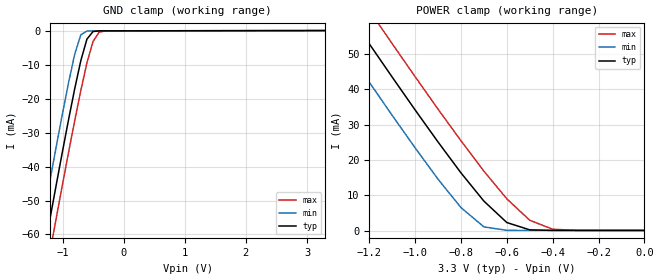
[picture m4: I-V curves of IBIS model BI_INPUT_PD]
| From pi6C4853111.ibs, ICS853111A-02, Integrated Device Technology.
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[Model]   BI_INPUT_PD
Model_type   Input
Polarity   Non-Inverting
Vinl = 1.4V
Vinh = 1.85V
|   typ   min   max
C_comp   2pF   1.5pF   2.5pF
|   typ   min   max
[Voltage range]  3.3V   3.15V   3.45V
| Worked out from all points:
|   GND clamp passes 1 mA (typ) near -0.54 V on its own axis
|   POWER clamp passes 1 mA (typ) near -0.54 V on its own axis
[GND_clamp]
|Voltage   I(typ)   I(min)   I(max)
-3.3V     -268.1mA   -256.8mA   -277.8mA
-1.4V     -74.7mA    -63.36mA   -84.54mA
-1.3V     -64.77mA   -53.44mA   -74.6mA
-1.2V     -54.9mA    -43.59mA   -64.73mA
-1.1V     -45.14mA   -33.87mA   -54.94mA
-800mV    -17.05mA   -6.868mA   -26.44mA
-700mV    -8.766mA   -1.163mA   -17.54mA
-600mV    -2.44mA    -56.74uA   -9.421mA
-500mV    -209.2uA   -18.47uA   -3.099mA
-400mV    -22.42uA   -15.4uA    -395.3uA
-300mV    -12.62uA   -12.97uA   -35.99uA
3.3V      69.2uA     64.69uA    70.79uA
[POWER_clamp]
|Voltage   I(typ)   I(min)   I(max)
-3.3V     258.1mA    247.7mA    267.2mA
-1.4V     71.88mA    61.05mA    81.34mA
-1.3V     62.31mA    51.46mA    71.78mA
-1.2V     52.81mA    41.96mA    62.27mA
-1.1V     43.4mA     32.58mA    52.84mA
-900mV    25.06mA    14.54mA    34.34mA
-800mV    16.33mA    6.517mA    25.4mA
-700mV    8.352mA    1.072mA    16.82mA
-600mV    2.299mA    101uA      9.001mA
-500mV    236.8uA    74.9uA     2.945mA
-400mV    83.48uA    72.53uA    412.8uA
0V        69.2uA     64.69uA    70.79uA
